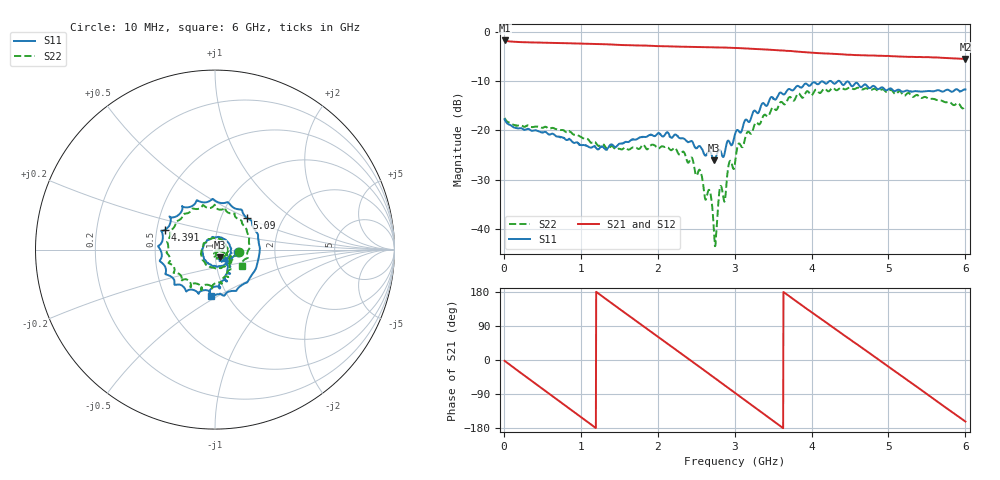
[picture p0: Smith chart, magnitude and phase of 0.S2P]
!Agilent Technologies,E5071C,MY46316741,A.11.02
!Date: Tue Oct 20 14:42:43 2020
!Data & Calibration Information:
!Freq	S11:SOLT4(ON)	S21:SOLT4(ON)	S12:SOLT4(ON)	S22:SOLT4(ON)
!PortZ  Port1:50+j0  Port2:50+j0
!Above PortZ is port z conversion or system Z0 setting when saving the data.
!When reading, reference impedance value at option line is always used.
# Hz S dB R 50
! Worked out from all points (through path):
!   1561 points, 10 MHz to 6 GHz, reference 50 ohm
!   highest |S21| = -1.76 dB at 10 MHz (marker M1); lowest = -5.5 dB at 6 GHz (marker M2)
!   group delay of S21, straight-line fit = 408 ps
!   lowest |S11| = -26.1 dB at 2.736 GHz (marker M3), VSWR 1.10, Z = 52.5 - j4.45 ohm
!   |S11| at or under -10 dB: start of sweep to 4.234 GHz; 4.251 GHz to 4.341 GHz (89.98 MHz wide, 2.09 % of centre); 4.364 GHz to end of sweep
!   |S22| runs from -43.5 to -11.3 dB; largest |S21 - S12| = 0.0059
!   S11 on the Smith chart (normalised r, x): 10 MHz: 1.30, -0.03; 4.391 GHz: 0.55, +0.14; 5.09 GHz: 1.33, +0.50; 6 GHz: 0.84, -0.47
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1e7  -17.75 -5.5  -1.76 -2.2  -1.80 -2.2  -17.48 -5.0
5.322051e8  -20.31 -81.6  -2.21 -80.5  -2.25 -80.5  -19.29 -70.6
7.5875e8  -21.44 -119.6  -2.30 -114.3  -2.32 -114.4  -19.90 -104.7
1.012173e9  -23.01 -169.7  -2.40 -152.1  -2.42 -152.2  -21.44 -148.7
1.288635e9  -23.37 128.8  -2.52 166.7  -2.53 166.7  -22.84 151.9
1.584295e9  -22.32 59.9  -2.70 123.0  -2.72 122.9  -23.56 79.5
2.006667e9  -20.55 -11.2  -2.91 60.7  -2.92 60.6  -23.67 -9.7
2.444397e9  -22.22 -60.2  -3.06 -3.5  -3.08 -3.9  -25.54 -77.3
2.678622e9  -24.20 -59.3  -3.14 -38.1  -3.16 -38.6  -32.38 -79.4
2.736218e9  -26.08 -58.5  -3.15 -46.8  -3.18 -47.0  -41.95 -40.9
2.813013e9  -24.06 -43.4  -3.17 -58.2  -3.22 -58.5  -31.40 -16.0
2.866769e9  -24.92 -50.4  -3.20 -66.3  -3.23 -66.5  -34.47 9.9
2.932045e9  -22.33 -38.4  -3.22 -76.0  -3.27 -76.3  -26.39 -5.9
3.005e9  -20.80 -47.7  -3.27 -87.0  -3.31 -87.2  -26.66 -15.3
3.527205e9  -13.77 -87.4  -3.70 -164.6  -3.73 -164.8  -15.79 -66.4
4.007173e9  -10.44 -152.0  -4.25 125.3  -4.26 125.1  -12.83 -132.9
4.391147e9  -10.51 158.1  -4.57 70.0  -4.59 69.7  -11.37 -177.0
4.709846e9  -10.77 109.4  -4.78 24.4  -4.82 24.2  -11.46 144.5
5.001667e9  -11.63 58.9  -4.90 -18.0  -4.94 -18.0  -12.05 107.3
5.089981e9  -12.01 44.5  -4.96 -30.7  -5.00 -30.7  -12.64 97.5
5.523872e9  -12.01 -26.9  -5.15 -93.3  -5.17 -93.3  -13.59 43.1
6e9  -11.71 -94.4  -5.52 -162.3  -5.51 -162.3  -14.98 -31.6
